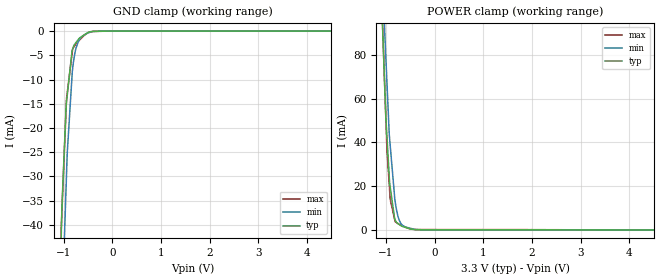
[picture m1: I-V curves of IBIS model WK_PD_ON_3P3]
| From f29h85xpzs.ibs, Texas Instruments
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|   Model Cell WK_PD_ON_3P3
|WK_PD_ON_3P3
[Model]   WK_PD_ON_3P3
Model_type   Input
Polarity   Non-Inverting
Vinl = 0.8
Vinh = 2
|   typ   min   max
C_comp   0.36pF   0.33pF   0.38pF
[Model Spec]
Vinl   0.8   0.8   0.8
Vinh   2   2   2
[Temperature Range]   25   155   -40
[Voltage Range]   3.3   2.8   3.63
| Nom Voltages:
|   VDD=1.23, VDDS=3.3, VSS=0
| Min Voltages:
|   VDD=1.08, VDDS=2.8, VSS=0
| Max Voltages:
|   VDD=1.32, VDDS=3.63, VSS=0
[Power Clamp Reference]   3.3   2.8   3.63
[GND Clamp Reference]   0   0   0
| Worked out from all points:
|   GND clamp passes 1 mA (typ) near -0.61 V on its own axis
|   POWER clamp passes 1 mA (typ) near -0.58 V on its own axis
[GND Clamp]
|   Voltage   I(typ)   I(min)   I(max)
-3.3V     -1.461A    -1.198A    -2.144A
-1.047V   -41.85mA   -64.11mA   -40.57mA
-1.024V   -33.99mA   -55.26mA   -34.89mA
-945.8mV  -15.2mA    -31.58mA   -15.49mA
-940mV    -14.67mA   -29.82mA   -14.04mA
-925.2mV  -13.3mA    -25.33mA   -12.83mA
-824.5mV  -4.036mA   -9.056mA   -4.623mA
-813.6mV  -3.713mA   -7.765mA   -3.735mA
-758mV    -2.545mA   -4.094mA   -2.814mA
-702.4mV  -1.801mA   -2.309mA   -2.152mA
-493.4mV  -249.4uA   -360.8uA   -341.5uA
6.6V      0A         0A         0A
[POWER Clamp]
|   Voltage   I(typ)   I(min)   I(max)
-3.3V     1.933A     2.239A     2.093A
-1.07V    91.57mA    120.8mA    92.54mA
-1.035V   70.43mA    95.89mA    70.73mA
-1.024V   63.33mA    88.73mA    63.41mA
-978.5mV  41.44mA    65.89mA    35.64mA
-934.4mV  24.29mA    43.67mA    20.58mA
-915.1mV  19.67mA    38.67mA    14mA
-819.6mV  5.013mA    13.9mA     4.441mA
-758mV    2.982mA    6.479mA    2.94mA
-687.9mV  1.839mA    2.781mA    2.125mA
-220.9mV  124.7uA    52.17uA    176.5uA
6.6V      0A         0A         0A
